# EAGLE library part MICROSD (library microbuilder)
MicroSD/Transflash Card Holder with SPI pinout 3M: 2908-05WB-MG 4UConnector: 19656 Footprint courtesy: Adafruit Industries
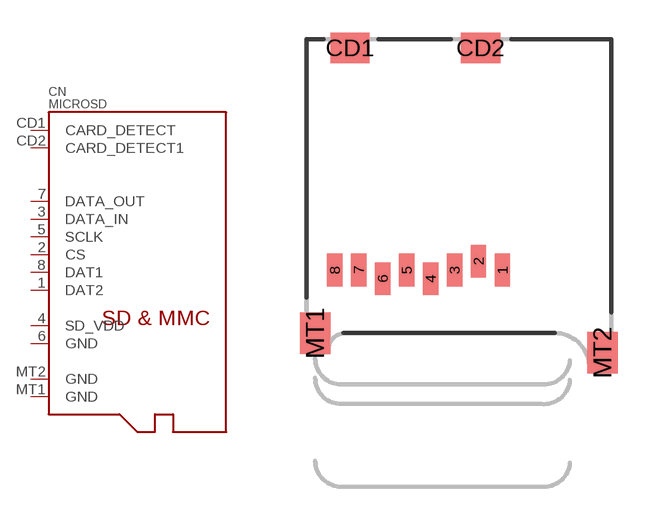
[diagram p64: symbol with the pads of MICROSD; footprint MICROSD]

Designator prefix CN

## MICROSD  [MICROSD]
1  DAT2
2  CS  in
3  DATA_IN  in
4  SD_VDD  pwr
5  SCLK  in
6  GND  pwr
7  DATA_OUT  out
8  DAT1
CD1  CARD_DETECT  pas
CD2  CARD_DETECT1  pas
MT1  GND  pwr
MT2  GND  pwr

## Footprint MICROSD (pad centres in mm)
Courtesy: Adafruit Industries
smd 0.7 x 1.5: 1 9,-10.64; 2 7.9,-10.24; 3 6.8,-10.64; 4 5.7,-11.04; 5 4.6,-10.64; 6 3.5,-11.04; 7 2.4,-10.64; 8 1.3,-10.64
smd 1.8 x 1.4: CD1 2,-0.44; CD2 8,-0.44
smd 1.4 x 1.9: MT1 0.4,-13.54; MT2 13.6,-14.44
